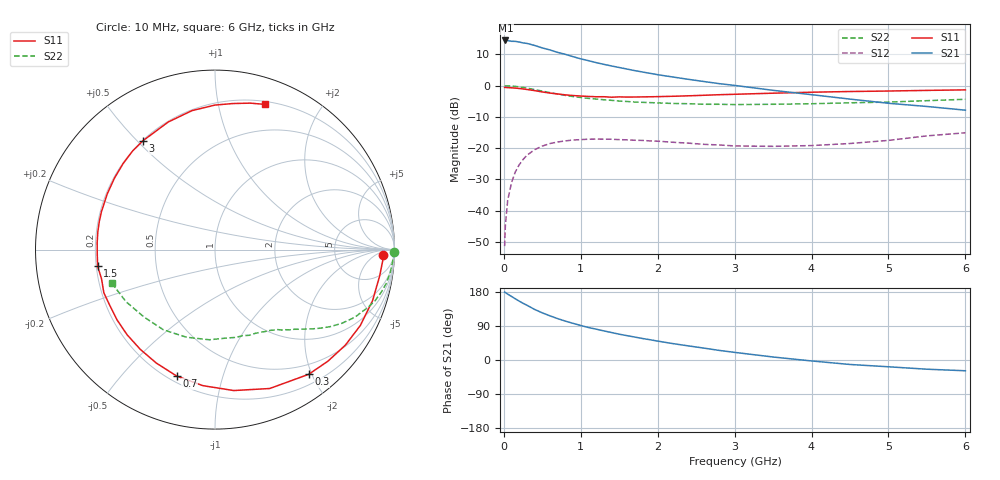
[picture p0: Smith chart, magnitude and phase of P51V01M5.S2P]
! SIEMENS Small Signal Semiconductors
! BFP183
! Si NPN RF Bipolar Junction Transistor in SOT143
! VCE = 1 V  IC = 1.5 mA
! Common Emitter S-Parameters:  March  1996
# GHz  S  MA  R  50
!  f  S11  S21  S12  S22
! GHz  MAG  ANG  MAG  ANG  MAG  ANG  MAG  ANG
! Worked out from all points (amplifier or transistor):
!   36 points, 10 MHz to 6 GHz, reference 50 ohm
!   highest |S21| = 14.5 dB at 20 MHz (marker M1)
!   |S21| within 3 dB of that: start of sweep to 593.6 MHz
!   unconditionally stable (mu >= 1): 2.183 GHz to end of sweep
!   at 250 MHz: K = 0.11, MSG = 18.7 dB, |S12| = -23.6 dB
!   at 1.4 GHz: K = 0.63, MSG = 11.7 dB, |S12| = -17.2 dB
!   at 6 GHz: K = 1.12, MAG = 1.5 dB, |S12| = -15.1 dB
!   S11 on the Smith chart (normalised r, x): 10 MHz: 25, -12; 300 MHz: 0.34, -1.95; 700 MHz: 0.23, -0.72; 1.5 GHz: 0.21, -0.07; 3 GHz: 0.20, +0.52; 6 GHz: 0.23, +1.38
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0.01  0.9378 -1.8  5.195 179.1  0.0027 87.4  0.999 -0.7
0.02  0.9365 -3.8  5.284 178.1  0.0058 90.7  0.9922 -1.5
0.05  0.9291 -9.1  5.266 173.8  0.0146 85.5  0.9923 -3.7
0.1  0.9229 -18.0  5.123 167.7  0.0281 78.6  0.9846 -7.4
0.15  0.9133 -27.6  5.111 161.4  0.0418 74.0  0.9729 -11.1
0.2  0.9006 -36.2  4.988 155.3  0.0542 69.1  0.956 -14.4
0.3  0.869 -53.1  4.738 144.5  0.0768 59.6  0.9129 -20.5
0.4  0.8318 -68.5  4.399 133.5  0.0945 51.0  0.8646 -25.9
0.5  0.7922 -82.4  4.013 124.4  0.1079 43.9  0.817 -30.2
0.6  0.761 -95.1  3.723 116.5  0.1186 37.6  0.7732 -33.7
0.7  0.7361 -106.9  3.402 109.2  0.1253 32.1  0.7324 -36.7
0.9  0.6944 -126.8  2.909 96.7  0.1348 23.4  0.6692 -41.4
1.1  0.6718 -144.4  2.51 85.7  0.1391 16.6  0.6256 -45.2
1.3  0.6645 -158.7  2.191 76.8  0.1393 11.0  0.5941 -48.7
1.5  0.6605 -171.9  1.951 68.1  0.1368 6.9  0.5664 -51.9
1.8  0.6603 171.3  1.655 56.8  0.1329 2.6  0.5407 -56.7
2.2  0.6759 152.6  1.373 43.2  0.1241 -0.9  0.518 -64.1
3  0.7273 123.5  1.009 20.1  0.1085 0.2  0.4974 -81.4
3.5  0.7572 110.1  0.841 7.9  0.1068 5.1  0.5033 -93.6
4.5  0.8053 90.0  0.609 -11.8  0.1186 15.0  0.5313 -122.7
5.5  0.8392 76.5  0.464 -24.3  0.1571 18.3  0.5747 -149.7
6  0.8557 71.0  0.405 -28.4  0.1761 15.5  0.6051 -162.1
